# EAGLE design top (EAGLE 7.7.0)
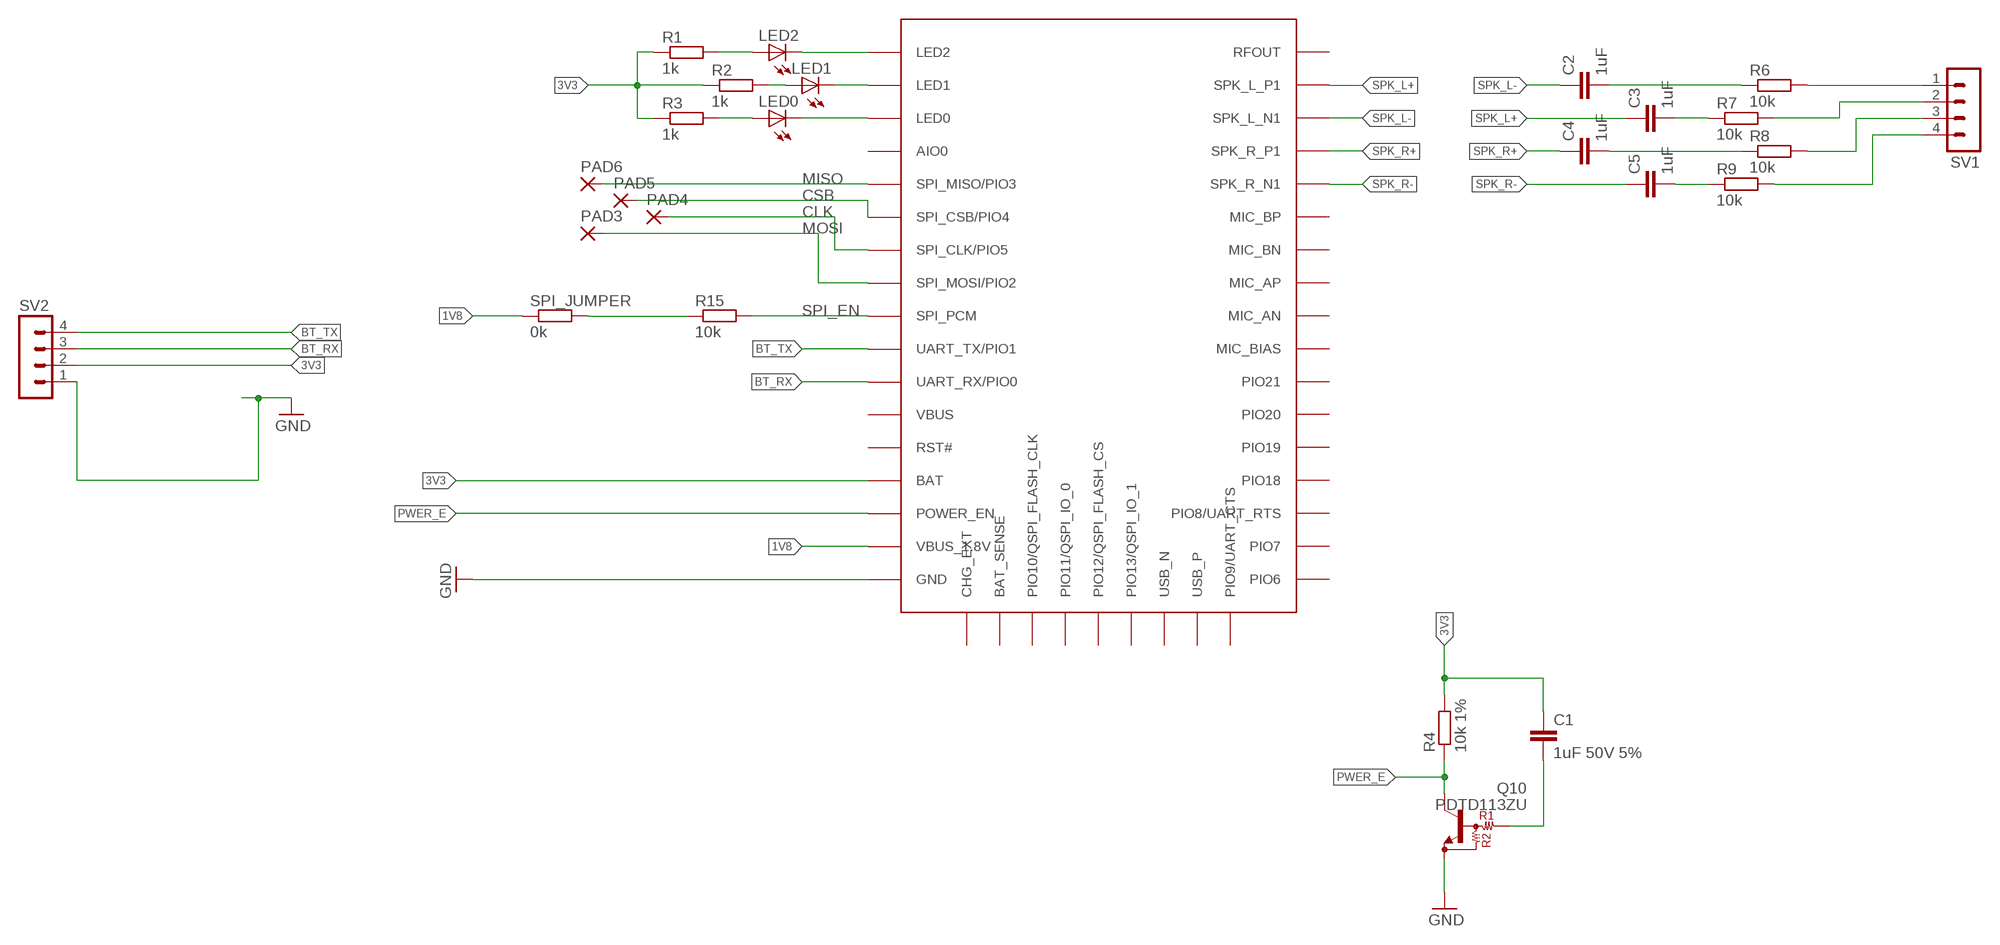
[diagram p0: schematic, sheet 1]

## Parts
C1  1uF 50V 5%  C-EUC0805  [C0805]
C2  1uF  C-EUC0805  [C0805]
C3  1uF  C-EUC0805  [C0805]
C4  1uF  C-EUC0805  [C0805]
C5  1uF  C-EUC0805  [C0805]
LED0  LEDSMART-LED  [SMART-LED]
LED1  LEDSMART-LED  [SMART-LED]
LED2  LEDSMART-LED  [SMART-LED]
PAD3  SMD2  [SMD1,27-2,54]
PAD4  SMD2  [SMD1,27-2,54]
PAD5  SMD2  [SMD1,27-2,54]
PAD6  SMD2  [SMD1,27-2,54]
Q10  PDTD113ZU  [SOT-23]
R1  1k  R-EU_R0805  [R0805]
R2  1k  R-EU_R0805  [R0805]
R3  1k  R-EU_R0805  [R0805]
R4  10k 1%  R-EU_R0805  [R0805]
R6  10k  R-EU_R0805  [R0805]
R7  10k  R-EU_R0805  [R0805]
R8  10k  R-EU_R0805  [R0805]
R9  10k  R-EU_R0805  [R0805]
R15  10k  R-EU_R0805  [R0805]
SPI_JUMPER  0k  R-EU_R0805  [R0805]
SV1  MA04-1  [MA04-1]
SV2  MA04-1  [MA04-1]
U$2  F3188-CSR8645-Good  F3188  [F3188]

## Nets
1V8: SPI_JUMPER.1 U$2.P$16(VBUS_1.8V)
3V3: C1.1 R1.1 R2.1 R3.1 R4.2 SV2.2 U$2.P$14(BAT)
BT_RX: SV2.3 U$2.P$11(UART_RX/PIO0)
BT_TX: SV2.4 U$2.P$10(UART_TX/PIO1)
CLK: PAD4.1(P) U$2.P$7(SPI_CLK/PIO5)
CSB: PAD5.1(P) U$2.P$6(SPI_CSB/PIO4)
GND: Q10.2(E) SV2.1 U$2.P$17(GND)
MISO: PAD6.1(P) U$2.P$5(SPI_MISO/PIO3)
MOSI: PAD3.1(P) U$2.P$8(SPI_MOSI/PIO2)
N$1: LED2.B(C) U$2.P$1(LED2)
N$2: LED1.B(C) U$2.P$2(LED1)
N$3: LED0.B(C) U$2.P$3(LED0)
N$4: LED2.A R1.2
N$5: LED1.A R2.2
N$6: LED0.A R3.2
N$7: R6.2 SV1.1
N$8: C2.2 R6.1
N$9: C1.2 Q10.1(B)
N$10: R7.2 SV1.2
N$11: C3.2 R7.1
N$12: R8.2 SV1.3
N$13: R9.2 SV1.4
N$14: C4.2 R8.1
N$15: C5.2 R9.1
N$16: R15.1 SPI_JUMPER.2
PWER_E: Q10.3(C) R4.1 U$2.P$15(POWER_EN)
SPI_EN: R15.2 U$2.P$9(SPI_PCM)
SPK_L+: C3.1 U$2.P$42(SPK_L_P1)
SPK_L-: C2.1 U$2.P$41(SPK_L_N1)
SPK_R+: C4.1 U$2.P$40(SPK_R_P1)
SPK_R-: C5.1 U$2.P$39(SPK_R_N1)
Unconnected: U$2.P$4(AIO0) U$2.P$13(RST#) U$2.P$18(CHG_EXT) U$2.P$19(BAT_SENSE) U$2.P$20(PIO10/QSPI_FLASH_CLK) U$2.P$21(PIO11/QSPI_IO_0) U$2.P$22(PIO12/QSPI_FLASH_CS) U$2.P$23(PIO13/QSPI_IO_1) U$2.P$24(USB_N) U$2.P$25(USB_P) U$2.P$26(PIO9/UART_CTS) U$2.P$27(PIO6) U$2.P$28(PIO7) U$2.P$29(PIO8/UART_RTS) U$2.P$30(PIO18) U$2.P$31(PIO19) U$2.P$32(PIO20) U$2.P$33(PIO21) U$2.P$34(MIC_BIAS) U$2.P$35(MIC_AN) U$2.P$36(MIC_AP) U$2.P$37(MIC_BN) U$2.P$38(MIC_BP) U$2.P$43(RFOUT)

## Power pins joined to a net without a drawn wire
VBUS: U$2.P$12(VBUS)

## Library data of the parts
C1 = resistor:C-EU: CAPACITOR, European symbol
C2-C5 = rcl:C-EU: CAPACITOR, European symbol
LED0 LED1 LED2 = led:LED: LED
PAD3-PAD6 = wirepad:SMD2: SMD PAD
Q10 = pre-bias-transistor:PDTD: Pre biase NPN transistor NPN Resistor-Equipped Transistor (RET) family in a very small SOT323 (SC-70) Surface-Mounted Device (SMD) plastic package. VCC = 50V Ic (max) = 500 mA; R1: 1 kOhm; R2: 10 kOhm
R1-R4 R6-R9 R15 SPI_JUMPER = resistor:R-EU_: RESISTOR, European symbol
SV1 SV2 = con-lstb:MA04-1: PIN HEADER; OC_FARNELL: unknown; OC_NEWARK: unknown
U$2 = f3188:F3188

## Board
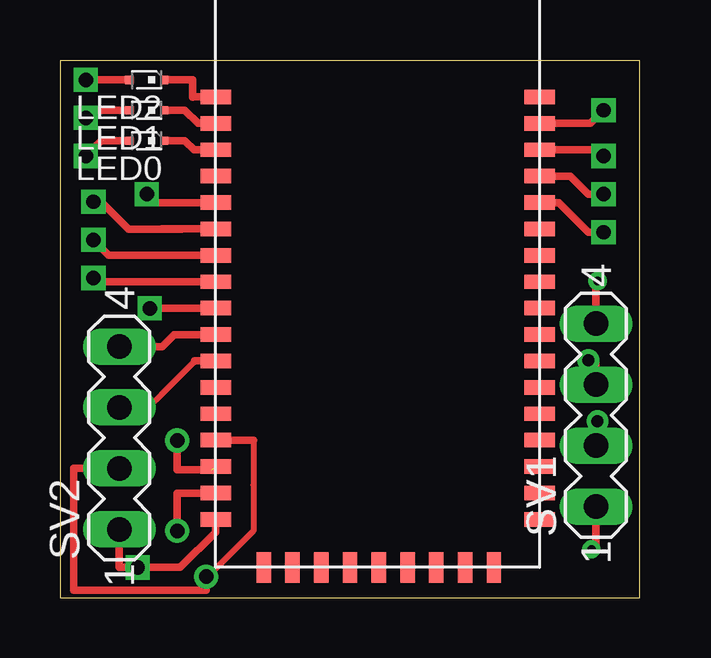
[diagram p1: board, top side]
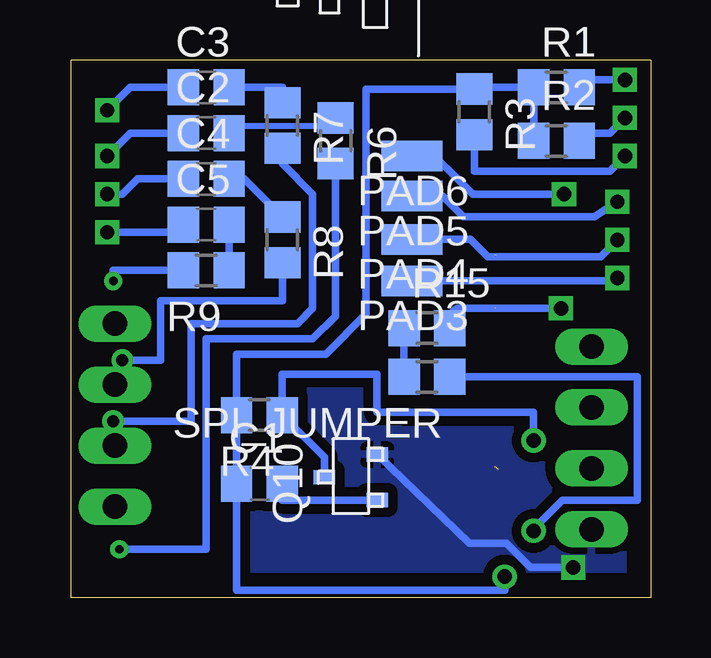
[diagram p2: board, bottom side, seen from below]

Size 24.17 x 22.42 mm. Coordinates in mm from the lower left corner, seen from the top.
Outline: 0,0 24.17,0 24.17,22.42 0,22.42 0,0
Copper layers (1*16): Top 0.035mm / dielectric 1.5mm / Bottom 0.035mm
Design rules "default": minimum track width 10mil, minimum drill 24mil, track to track 8mil, track to pad 8mil, pad to pad 8mil, via to via 8mil, smd to smd 8mil, copper to edge 40mil, drill to drill 8mil, minimum pad ring 10mil, minimum via ring 8mil, stop-mask expansion 4mil, vias tented up to drill 0mil, thermal gap 10mil

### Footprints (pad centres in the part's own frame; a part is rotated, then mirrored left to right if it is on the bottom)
C0805 = smd 1.3 x 1.5: 1 -0.95,0; 2 0.95,0
SMART-LED = smd 0.35 x 0.35: A 0,0.725; B 0,-0.725
SMD1,27-2,54 = smd 1.27 x 2.54: 1 0,0
SOT-23 = smd 0.6 x 0.9: 1 -1,-1.1; 2 0.9,-1.1; 3 -0.05,1.1
R0805 = smd 1.3 x 1.5: 1 -0.95,0; 2 0.95,0
MA04-1 = drill 1.016 long: 1 -3.81,0; 2 -1.27,0; 3 1.27,0; 4 3.81,0
F3188 = smd 1.27 x 0.6: P$1 -6.5,7.7; P$2 -6.5,6.6; P$3 -6.5,5.5; P$4 -6.5,4.4; P$5 -6.5,3.3; P$6 -6.5,2.2; P$7 -6.5,1.1; P$8 -6.5,0; P$9 -6.5,-1.1; P$10 -6.5,-2.2; P$11 -6.5,-3.3; P$12 -6.5,-4.4; P$13 -6.5,-5.5; P$14 -6.5,-6.6; P$15 -6.5,-7.7; P$16 -6.5,-8.8; P$17 -6.5,-9.9; P$27 7,-9.9; P$28 7,-8.8; P$29 7,-7.7; P$30 7,-6.6; P$31 7,-5.5; P$32 7,-4.4; P$33 7,-3.3; P$34 7,-2.2; P$35 7,-1.1; P$36 7,0; P$37 7,1.1; P$38 7,2.2; P$39 7,3.3; P$40 7,4.4; P$41 7,5.5; P$42 7,6.6; P$43 7,7.7 | smd 0.6 x 1.27: P$18 -4.5,-11.9; P$19 -3.3,-11.9; P$20 -2.1,-11.9; P$21 -0.9,-11.9; P$22 0.3,-11.9; P$23 1.5,-11.9; P$24 2.7,-11.9; P$25 3.9,-11.9; P$26 5.1,-11.9

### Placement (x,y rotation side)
C1  16.32,4.76 0 bottom
C2  18.54,19.37 0 bottom
C3  18.54,21.27 0 bottom
C4  18.54,17.46 0 bottom
C5  18.54,15.56 0 bottom
LED0  3.62,19.05 90 top
LED1  3.62,20.32 90 top
LED2  3.62,21.59 90 top
PAD3  9.97,13.21 90 bottom
PAD4  9.97,14.94 90 bottom
PAD5  9.97,16.74 90 bottom
PAD6  9.97,18.41 90 bottom
Q10  12.51,5.08 90 bottom
R1  3.94,21.27 0 bottom
R2  3.94,19.05 0 bottom
R3  7.37,20.26 270 bottom
R4  16.32,7.62 180 bottom
R6  13.14,19.05 270 bottom
R7  15.37,19.69 270 bottom
R8  15.37,14.92 270 bottom
R9  18.54,13.65 180 bottom
R15  9.33,11.24 0 bottom
SPI_JUMPER  9.33,9.21 180 bottom
SV1  22.35,7.62 90 top
SV2  2.48,6.67 90 top
U$2  12.99,13.17 0 top

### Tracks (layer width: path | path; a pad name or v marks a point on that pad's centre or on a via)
1V8  (via drill 0.6)
  Top 0.305: v4.89,2.79 4.89,4.37 U$2.P$16
  Bottom 0.305: SPI_JUMPER.1 5.84,9.21 0.57,9.21 0.57,7.94 0.57,4.06 1.08,4.06 2.98,4.06 3.68,4.06 4.89,2.86 v4.89,2.79
3V3  (via drill 0.6)
  Top 0.254: 8.06,6.57 8.06,4.7 8.06,2.79 6.16,0.89 v6.1,0.89
  Top 0.305: v6.1,0.89 6.1,0.32 0.57,0.32 0.57,4.13 0.57,5.4 SV2.2 | U$2.P$14 8.06,6.57
  Bottom 0.305: v6.1,0.89 6.1,0.32 17.27,0.32 C1.1 R4.2 17.27,10.16 14.41,10.16 13.55,10.16 11.87,11.84 11.87,20.64 11.87,21.21 R3.1 7.3,21.27 R1.1 R2.1
BT_RX
  Top 0.254: 5.62,9.87 4.25,8.51 3.68,7.94 SV2.3
  Top 0.305: U$2.P$11 5.62,9.87
BT_TX
  Top 0.305: SV2.4 4.25,10.48 4.75,10.97 U$2.P$10
CLK  (via drill 0.6)  (1 unrouted)
  Top 0.305: 6.46,14.29 4.89,14.29 2.03,14.29 v1.4,14.92
  Bottom 0.305: v1.4,14.92 2.1,14.22 6.79,14.22 7.51,14.94 PAD4.1
CSB  (via drill 0.6)
  Top 0.305: 4.25,15.37 2.85,15.37 1.71,16.51 v1.4,16.51 | 4.25,15.37 5.08,15.37 | U$2.P$6 4.26,15.37 4.25,15.37
  Bottom 0.305: v1.4,16.51 2.35,15.88 3.62,15.88 7.11,15.88 7.81,15.88 8.06,16.13 8.68,16.74 PAD5.1
GND  (via drill 0.6)
  Top 0.305: SV2.1 2.48,1.27 v3.24,1.27 5.02,1.27 6.49,2.75 U$2.P$17
  Bottom 0.305: Q10.2 7.56,2.29 6.03,2.29 5.14,1.4 5.02,1.27 v3.24,1.27
  pour Bottom (isolate 0.406): 25.84,22.86 -0.83,22.86 -0.83,-1.27 25.84,-1.27
MISO  (via drill 0.6)
  Top 0.305: v3.62,16.83 3.98,16.47 5.25,16.47 U$2.P$5
  Bottom 0.305: v3.62,16.83 7.43,16.83 8.06,17.46 9.02,18.41 PAD6.1
MOSI  (via drill 0.6)
  Top 0.305: v1.4,13.34 1.4,13.17 4.42,13.17 U$2.P$8
  Bottom 0.305: PAD3.1 5.02,13.21 1.4,13.21 v1.4,13.34
N$1
  Top 0.305: LED2.B 5.52,21.59 5.52,20.87 5.53,20.87 U$2.P$1
N$2
  Top 0.305: 4.77,20.32 LED1.B 5.21,20.32 5.76,19.77 U$2.P$2
N$3
  Top 0.305: LED0.B 5.21,19.05 5.59,18.67 U$2.P$3
N$4  (via drill 0.6)
  Top 0.305: LED2.A v1.08,21.59
  Bottom 0.305: v1.08,21.59 2.67,21.59 R1.2
N$5  (via drill 0.6)
  Top 0.305: LED1.A 1.4,20.32 v1.08,20
  Bottom 0.305: R2.2 2.99,19.37 1.71,19.37 v1.08,20
N$6  (via drill 0.6)
  Top 0.305: LED0.A 1.71,19.05 v1.08,18.41
  Bottom 0.305: v1.08,18.41 1.71,17.78 2.98,17.78 7.37,17.78 R3.2
N$7  (via drill 0.35)
  Top 0.305: SV1.1 22.35,2.22 arc-90 v22.16,2.03
  Bottom 0.305: R6.2 13.14,11.75 14.1,10.79 18.54,10.79 18.54,2.03 v22.16,2.03
N$8
  Bottom 0.254: 17.27,19.69 13.46,19.69
  Bottom 0.305: C2.2 17.27,19.69 | 13.46,19.69 R6.1
N$9
  Bottom 0.305: C1.2 15.37,4.08 Q10.1
N$10  (via drill 0.5)
  Top 0.305: v22.42,7.37 22.35,7.37 SV1.2
  Bottom 0.305: R7.2 15.37,18.1 14.1,16.83 14.1,12.07 14.73,11.43 19.18,11.43 19.18,7.37 v22.42,7.37
N$11
  Bottom 0.305: C3.2 15.37,21.27 R7.1
N$12  (via drill 0.5)
  Top 0.305: SV1.3 22.35,9.91 v22.03,9.91
  Bottom 0.305: R8.2 15.37,12.38 20.45,12.38 20.45,9.91 v22.03,9.91 22.29,9.91
N$13  (via drill 0.35)
  Top 0.305: v22.42,13.21 arc90 22.35,13.14 SV1.4
  Bottom 0.305: R9.2 22.42,13.65 v22.42,13.21
N$14
  Bottom 0.305: C4.2 16.96,17.46 R8.1
N$15
  Bottom 0.305: C5.2 R9.1
N$16
  Bottom 0.305: R15.1 10.28,9.31 SPI_JUMPER.2
PWER_E  (via drill 0.6)  (1 unrouted)
  Top 0.305: v4.89,6.56 4.89,5.33 6.34,5.33
  Bottom 0.305: v4.89,6.56 4.89,7.75 10.35,7.75 11.42,7.75 11.42,9.32 15.37,9.32 R4.1 13.61,5.86 Q10.3
SPI_EN  (via drill 0.6)  (1 unrouted)
  Top 0.305: 6.47,12.07 v3.75,12.07
  Bottom 0.305: R15.2 arc90 8.07,12.07 v3.75,12.07
SPK_L+  (via drill 0.6)
  Top 0.305: v22.67,20.32 22.12,19.77 U$2.P$42
  Bottom 0.305: C3.1 21.72,21.27 v22.67,20.32
SPK_L-  (via drill 0.6)
  Top 0.305: 22.41,18.67 v22.67,18.41 22.41,18.67 U$2.P$41
  Bottom 0.305: C2.1 21.72,19.37 v22.67,18.41
SPK_R+  (via drill 0.6)
  Top 0.305: v22.67,16.83 22.03,16.83 21.29,17.57 U$2.P$40
  Bottom 0.305: C4.1 21.4,17.46 22.03,16.83 v22.67,16.83
SPK_R-  (via drill 0.6)
  Top 0.305: v22.67,15.24 22.03,15.24 20.8,16.47 U$2.P$39
  Bottom 0.305: C5.1 19.49,15.88 20.13,15.24 v22.67,15.24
